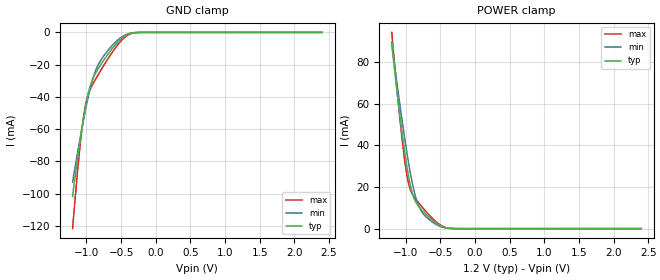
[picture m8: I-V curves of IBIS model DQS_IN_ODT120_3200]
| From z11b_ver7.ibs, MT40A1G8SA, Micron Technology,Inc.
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| MODEL DQS_IN_ODT120_3200 (Data Strobe Input with 120ohm ODT, 1600-3200Mbps)
[Model]   DQS_IN_ODT120_3200
Model_type   Input
Vinl = 905.000mV
Vinh = 1015.000mV
|   typ   min   max
|C_comp   0.801pF   0.748pF   0.856pF
C_comp_power_clamp   0.4005pF   0.3740pF   0.4280pF
C_comp_gnd_clamp   0.4005pF   0.3740pF   0.4280pF
| Note: C_comp changes when the ODT circuit is enabled.
|[Model Spec]
| Dynamic Overshoot Parameters from DDR4 Specification
|D_overshoot_ampl_h   0.40   NA   NA
|D_overshoot_ampl_l   0.40   NA   NA
|D_overshoot_area_h   0.0800n   NA   NA
|D_overshoot_area_l   0.0800n   NA   NA
[Voltage Range]   1.2000V   1.1400V   1.2600V
| Junction Temperature (Ambient temp is 35C typ, 95C min, 0C max)
[Temperature Range]   50.0   110.0   0.0
[Add Submodel]
| Submodel Name   Mode
120ohm_ODT_3200   Non-Driving
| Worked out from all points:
|   GND clamp passes 1 mA (typ) near -0.39 V on its own axis
|   POWER clamp passes 1 mA (typ) near -0.48 V on its own axis
[GND_clamp]
|   Voltage   I(typ)   I(min)   I(max)
-1.2V     -101.7mA   -92.84mA   -121.7mA
-1.135V   -79.96mA   -75.84mA   -88.92mA
-1.08V    -63.49mA   -62.76mA   -65.41mA
-1.036V   -51.56mA   -52.83mA   -50.65mA
-992.7mV  -41.38mA   -43.57mA   -41.02mA
-927.3mV  -30.76mA   -31.6mA    -33.57mA
-872.7mV  -25.55mA   -24.13mA   -29.29mA
-818.2mV  -21.61mA   -19.01mA   -25.29mA
-621.8mV  -9.66mA    -7.8mA     -11.96mA
-436.4mV  -1.915mA   -1.476mA   -2.607mA
-229.1mV  -17.62uA   -20.1uA    -21.35uA
2.4V      0A         0A         0A
[POWER_clamp]
|   Voltage   I(typ)   I(min)   I(max)
-1.2V     88.79mA    89.61mA    94.2mA
-1.135V   68.71mA    72.12mA    70.03mA
-1.058V   47.63mA    53.55mA    44.95mA
-1.004V   34.46mA    41.11mA    30.27mA
-960mV    25.41mA    31.92mA    21.99mA
-894.5mV  16.02mA    20.41mA    16.03mA
-850.9mV  12.63mA    14.54mA    13.97mA
-807.3mV  10.5mA     10.53mA    12.15mA
-709.1mV  6.91mA     5.769mA    8.279mA
-545.5mV  2.224mA    1.735mA    2.842mA
-305.5mV  24.75uA    26.66uA    31.49uA
2.4V      0A         0A         0A
